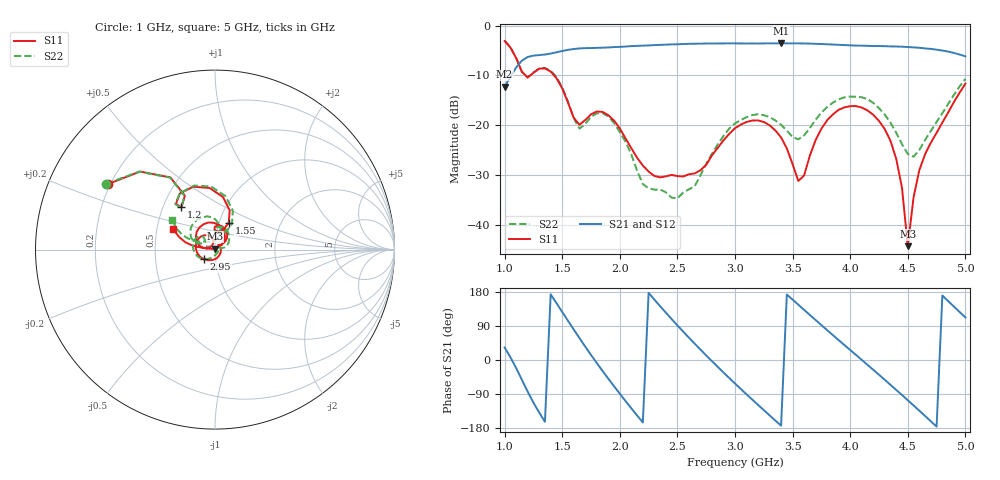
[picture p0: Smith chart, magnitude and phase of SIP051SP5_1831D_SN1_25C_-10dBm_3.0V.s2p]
# GHz  S  dB  R  50
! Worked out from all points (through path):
!   81 points, 1 GHz to 5 GHz, reference 50 ohm
!   highest |S21| = -3.56 dB at 3.4 GHz (marker M1); lowest = -12.3 dB at 1 GHz (marker M2)
!   lowest |S11| = -44.3 dB at 4.5 GHz (marker M3), VSWR 1.01, Z = 50.1 + j0.605 ohm
!   |S11| at or under -10 dB: 1.181 GHz to 1.224 GHz (42.39 MHz wide, 3.53 % of centre); 1.428 GHz to end of sweep
!   |S22| runs from -34.7 to -3.0 dB; largest |S21 - S12| = 0.0046
!   S11 on the Smith chart (normalised r, x): 1 GHz: 0.19, +0.27; 1.2 GHz: 0.62, +0.32; 1.55 GHz: 1.11, +0.34; 2.95 GHz: 0.88, -0.09; 5 GHz: 0.61, +0.15
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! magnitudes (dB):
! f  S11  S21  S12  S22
! 1 GHz  -3.1  -12.3  -12.2  -3.0
! 1.2 GHz  -10.4  -6.3  -6.3  -10.4
! 1.4 GHz  -9.2  -5.6  -5.6  -9.1
! 1.55 GHz  -15.5  -4.9  -4.9  -15.3
! 1.65 GHz  -19.9  -4.6  -4.6  -20.7
! 1.7 GHz  -19.0  -4.5  -4.6  -19.8
! 1.9 GHz  -18.0  -4.4  -4.4  -18.2
! 2.2 GHz  -28.1  -4.0  -4.0  -31.8
! 2.35 GHz  -30.5  -3.9  -3.9  -32.9
! 2.65 GHz  -29.7  -3.7  -3.7  -32.3
! 2.95 GHz  -21.8  -3.6  -3.6  -20.7
! 3 GHz  -20.6  -3.6  -3.6  -19.7
! 3.2 GHz  -19.1  -3.6  -3.6  -17.8
! 3.4 GHz  -22.5  -3.6  -3.6  -19.9
! 3.55 GHz  -31.2  -3.6  -3.6  -22.9
! 3.7 GHz  -23.0  -3.7  -3.7  -18.9
! 4.05 GHz  -16.2  -4.0  -4.0  -14.3
! 4.35 GHz  -23.2  -4.2  -4.2  -19.5
! 4.45 GHz  -32.6  -4.2  -4.3  -23.8
! 4.5 GHz  -44.3  -4.3  -4.3  -25.8
! 4.6 GHz  -29.1  -4.5  -4.5  -25.0
! 5 GHz  -11.7  -6.2  -6.2  -10.7
